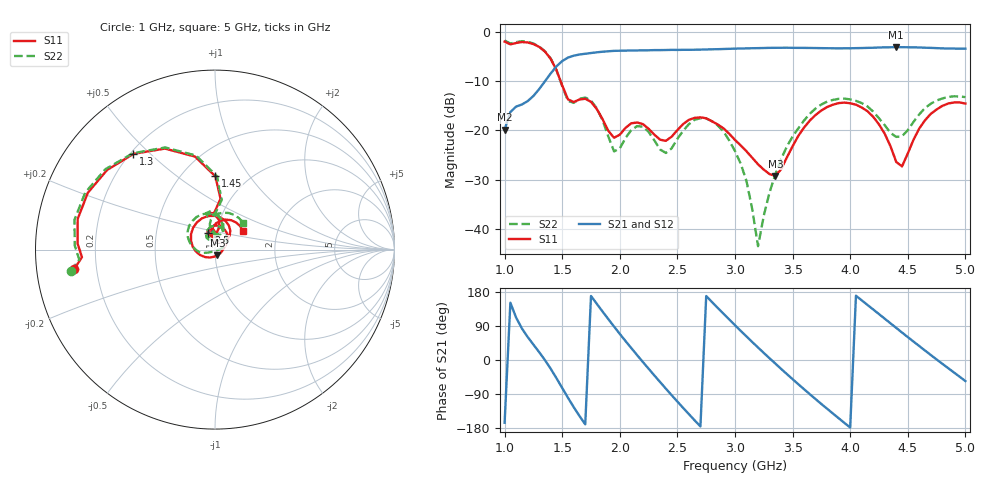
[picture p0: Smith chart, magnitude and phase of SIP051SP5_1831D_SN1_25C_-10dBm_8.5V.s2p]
# GHz  S  dB  R  50
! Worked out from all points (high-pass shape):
!   81 points, 1 GHz to 5 GHz, reference 50 ohm
!   highest |S21| = -3.14 dB at 4.4 GHz (marker M1); lowest = -19.9 dB at 1 GHz (marker M2)
!   |S21| within 3 dB of the highest: 1.492 GHz to end of sweep
!   lowest |S11| = -29.2 dB at 3.35 GHz (marker M3), VSWR 1.07, Z = 51.3 - j3.26 ohm
!   |S11| at or under -10 dB: 1.486 GHz to end of sweep
!   |S22| runs from -43.5 to -1.8 dB; largest |S21 - S12| = 0.0021
!   S11 on the Smith chart (normalised r, x): 1 GHz: 0.12, -0.07; 1.3 GHz: 0.21, +0.44; 1.45 GHz: 0.72, +0.70; 2.5 GHz: 0.91, +0.17; 5 GHz: 1.33, +0.29
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1  -2.03 -172.2  -19.87 -165.5  -19.88 -165.7  -1.79 -171.6
1.3  -3.09 130.4  -11.64 20.8  -11.65 20.9  -3.03 130.4
1.45  -7.79 89.7  -7.05 -47.9  -7.04 -47.8  -7.77 88.4
1.55  -13.72 91.1  -5.26 -99.6  -5.26 -99.6  -14.02 90.0
1.7  -13.61 97.8  -4.49 -169.8  -4.48 -169.8  -13.35 97.1
1.8  -15.68 82.0  -4.20 148.3  -4.20 148.4  -15.51 77.2
1.95  -21.50 97.0  -3.90 88.3  -3.91 88.3  -24.28 90.7
2.15  -18.41 102.6  -3.81 12.9  -3.82 13.0  -19.14 105.6
2.35  -21.90 95.8  -3.75 -58.2  -3.74 -58.2  -23.89 93.0
2.5  -19.95 111.6  -3.71 -109.7  -3.71 -109.7  -21.72 125.5
2.75  -17.56 72.8  -3.62 168.8  -3.62 168.9  -17.61 82.0
3  -21.95 33.8  -3.45 91.8  -3.45 91.9  -24.20 27.8
3.1  -24.25 20.8  -3.40 62.1  -3.39 62.1  -30.29 6.0
3.2  -26.88 2.9  -3.35 33.0  -3.35 33.1  -43.46 -69.8
3.35  -29.23 -66.6  -3.29 -9.4  -3.29 -9.3  -28.93 -154.1
3.55  -21.10 -159.9  -3.29 -64.0  -3.27 -64.0  -19.57 -178.7
3.7  -16.88 159.2  -3.33 -103.4  -3.33 -103.3  -15.57 155.4
4  -14.51 90.9  -3.38 -178.2  -3.38 -178.1  -13.73 101.6
4.35  -23.23 39.4  -3.17 96.8  -3.17 96.8  -20.52 72.4
4.4  -26.41 51.3  -3.14 84.7  -3.15 84.7  -21.33 82.1
4.7  -16.65 87.7  -3.30 13.2  -3.29 13.3  -14.60 92.3
5  -14.57 33.5  -3.45 -55.6  -3.46 -55.4  -13.27 43.7
